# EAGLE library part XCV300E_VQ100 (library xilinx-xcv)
xcv300e_vq100 edit this description Auto generated by make-symbol-device-package-bsdl.ulp Rev. 26 Source: xcv300e_vq100.bsd
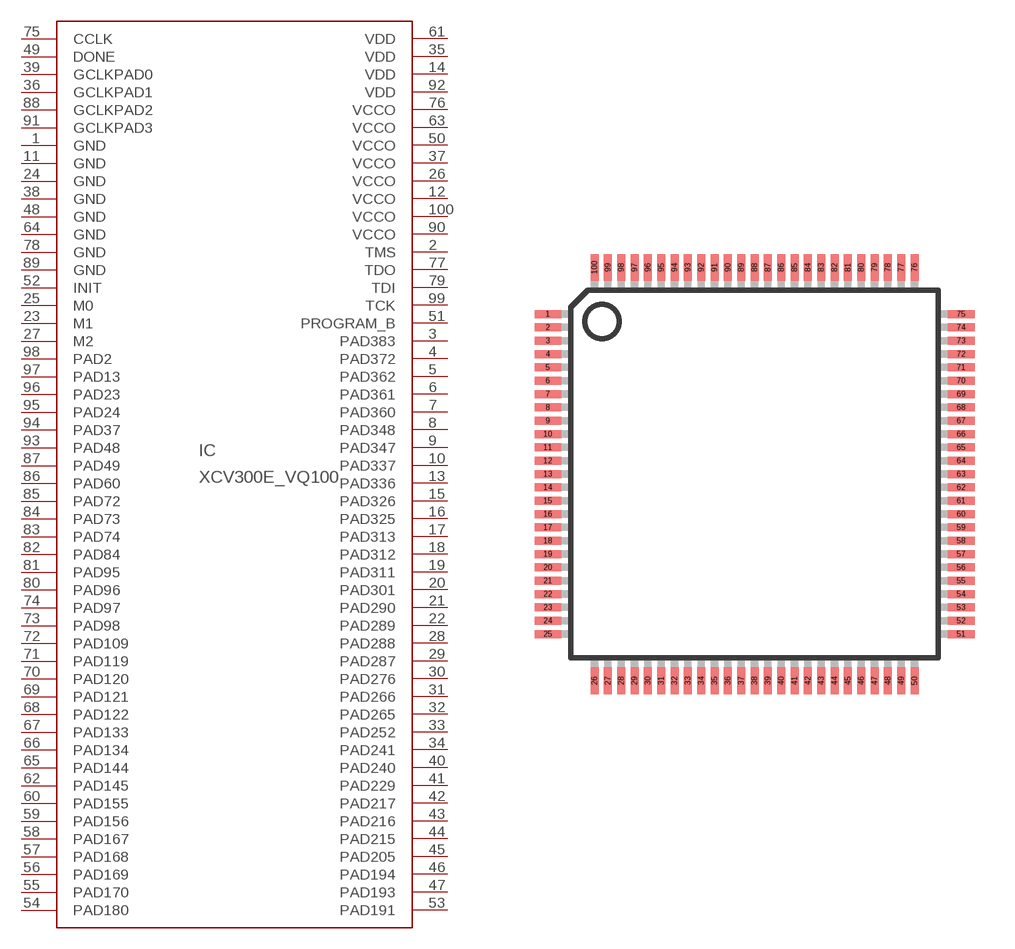
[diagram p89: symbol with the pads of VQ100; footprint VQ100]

Designator prefix IC

## XCV300E_VQ100 (OC_FARNELL: unknown; OC_NEWARK: unknown)  [VQ100]
1  GND  pwr
2  TMS  in
3  PAD383
4  PAD372
5  PAD362
6  PAD361
7  PAD360
8  PAD348
9  PAD347
10  PAD337
11  GND  pwr
12  VCCO  pwr
13  PAD336
14  VDD  pwr
15  PAD326
16  PAD325
17  PAD313
18  PAD312
19  PAD311
20  PAD301
21  PAD290
22  PAD289
23  M1  in
24  GND  pwr
25  M0  in
26  VCCO  pwr
27  M2  in
28  PAD288
29  PAD287
30  PAD276
31  PAD266
32  PAD265
33  PAD252
34  PAD241
35  VDD  pwr
36  GCLKPAD1  in
37  VCCO  pwr
38  GND  pwr
39  GCLKPAD0  in
40  PAD240
41  PAD229
42  PAD217
43  PAD216
44  PAD215
45  PAD205
46  PAD194
47  PAD193
48  GND  pwr
49  DONE
50  VCCO  pwr
51  PROGRAM_B  in
52  INIT
53  PAD191
54  PAD180
55  PAD170
56  PAD169
57  PAD168
58  PAD167
59  PAD156
60  PAD155
61  VDD  pwr
62  PAD145
63  VCCO  pwr
64  GND  pwr
65  PAD144
66  PAD134
67  PAD133
68  PAD122
69  PAD121
70  PAD120
71  PAD119
72  PAD109
73  PAD98
74  PAD97
75  CCLK
76  VCCO  pwr
77  TDO  out
78  GND  pwr
79  TDI  in
80  PAD96
81  PAD95
82  PAD84
83  PAD74
84  PAD73
85  PAD72
86  PAD60
87  PAD49
88  GCLKPAD2  in
89  GND  pwr
90  VCCO  pwr
91  GCLKPAD3  in
92  VDD  pwr
93  PAD48
94  PAD37
95  PAD24
96  PAD23
97  PAD13
98  PAD2
99  TCK  in
100  VCCO  pwr

## Footprint VQ100 (pad centres in mm)
VQ100 Auto generated by make-symbol-device-package-bsdl.ulp Rev. 26
smd 1 x 0.3: 1 -7.75,6; 2 -7.75,5.5; 3 -7.75,5; 4 -7.75,4.5; 5 -7.75,4; 6 -7.75,3.5; 7 -7.75,3; 8 -7.75,2.5; 9 -7.75,2; 10 -7.75,1.5; 11 -7.75,1; 12 -7.75,0.5; 13 -7.75,0; 14 -7.75,-0.5; 15 -7.75,-1; 16 -7.75,-1.5; 17 -7.75,-2; 18 -7.75,-2.5; 19 -7.75,-3; 20 -7.75,-3.5; 21 -7.75,-4; 22 -7.75,-4.5; 23 -7.75,-5; 24 -7.75,-5.5; 25 -7.75,-6; 51 7.75,-6; 52 7.75,-5.5; 53 7.75,-5; 54 7.75,-4.5; 55 7.75,-4; 56 7.75,-3.5; 57 7.75,-3; 58 7.75,-2.5; 59 7.75,-2; 60 7.75,-1.5; 61 7.75,-1; 62 7.75,-0.5; 63 7.75,0; 64 7.75,0.5; 65 7.75,1; 66 7.75,1.5; 67 7.75,2; 68 7.75,2.5; 69 7.75,3; 70 7.75,3.5; 71 7.75,4; 72 7.75,4.5; 73 7.75,5; 74 7.75,5.5; 75 7.75,6
smd 0.3 x 1: 26 -6,-7.75; 27 -5.5,-7.75; 28 -5,-7.75; 29 -4.5,-7.75; 30 -4,-7.75; 31 -3.5,-7.75; 32 -3,-7.75; 33 -2.5,-7.75; 34 -2,-7.75; 35 -1.5,-7.75; 36 -1,-7.75; 37 -0.5,-7.75; 38 0,-7.75; 39 0.5,-7.75; 40 1,-7.75; 41 1.5,-7.75; 42 2,-7.75; 43 2.5,-7.75; 44 3,-7.75; 45 3.5,-7.75; 46 4,-7.75; 47 4.5,-7.75; 48 5,-7.75; 49 5.5,-7.75; 50 6,-7.75; 76 6,7.75; 77 5.5,7.75; 78 5,7.75; 79 4.5,7.75; 80 4,7.75; 81 3.5,7.75; 82 3,7.75; 83 2.5,7.75; 84 2,7.75; 85 1.5,7.75; 86 1,7.75; 87 0.5,7.75; 88 0,7.75; 89 -0.5,7.75; 90 -1,7.75; 91 -1.5,7.75; 92 -2,7.75; 93 -2.5,7.75; 94 -3,7.75; 95 -3.5,7.75; 96 -4,7.75; 97 -4.5,7.75; 98 -5,7.75; 99 -5.5,7.75; 100 -6,7.75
